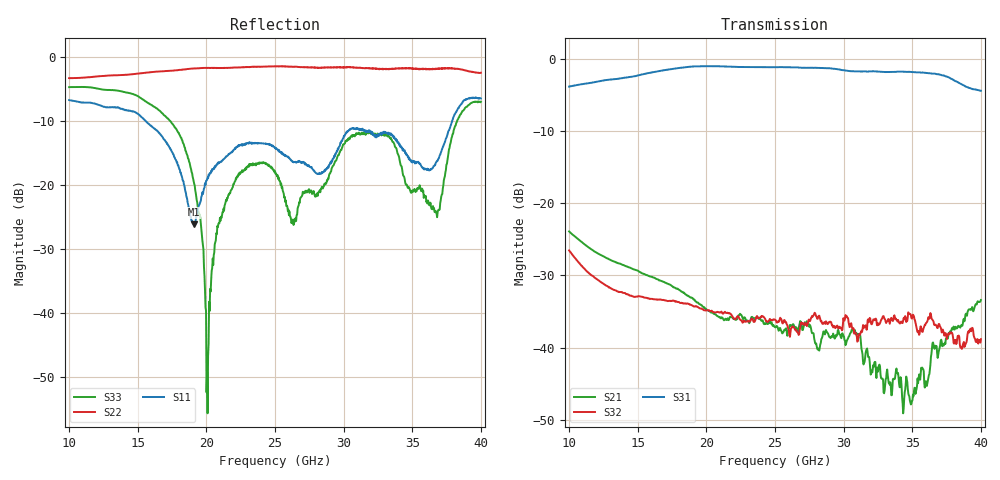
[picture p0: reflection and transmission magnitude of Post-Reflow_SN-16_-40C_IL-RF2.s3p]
!Agilent Technologies,N5245A,US49150155,A.09.90.19
!Agilent N5245A: A.09.90.19
!Date: Wednesday, November 14, 2018 00:01:03
!Correction: S11(Full 3 Port(1,2,3))
!S12(Full 3 Port(1,2,3))
!S13(Full 3 Port(1,2,3))
!S21(Full 3 Port(1,2,3))
!S22(Full 3 Port(1,2,3))
!S23(Full 3 Port(1,2,3))
!S31(Full 3 Port(1,2,3))
!S32(Full 3 Port(1,2,3))
!S33(Full 3 Port(1,2,3))
!S3P File: Measurements: <S11,S12,S13>,
!<S21,S22,S23>,
!<S31,S32,S33>:
# Hz S  dB  R 50
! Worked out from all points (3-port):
!   801 points, 10 GHz to 40 GHz, reference 50 ohm
!   strongest paths, dB at 10 GHz, 17.5 GHz, 25 GHz, 32.5 GHz, 40 GHz:
!     S31: -3.9, -1.4, -1.2, -1.8, -4.4
!     S32: -26.6, -33.5, -36.1, -36.6, -38.8
!     S21: -23.9, -31.5, -37.2, -43.3, -33.4
!   lowest |S11| = -26.2 dB at 19.11 GHz (marker M1), VSWR 1.10, Z = 45.5 - j1.2 ohm
!   |S11| at or under -10 dB: 15.59 GHz to 37.9 GHz (22.31 GHz wide, 83.4 % of centre)
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1e10  -6.70 -5.9  -23.93 59.2  -3.87 -169.8
      -23.93 59.4  -3.27 51.8  -26.57 -6.4
      -3.87 -169.6  -26.55 -6.2  -4.68 -116.9
1.49125e10  -8.70 -156.0  -29.29 -30.0  -2.38 78.0
            -29.30 -29.9  -2.58 -54.0  -32.98 -89.2
            -2.38 78.2  -32.96 -89.1  -5.99 147.9
1.91125e10  -26.15 -164.5  -33.38 -111.6  -1.08 -22.5
            -33.34 -111.5  -1.75 -126.6  -34.33 176.7
            -1.08 -22.3  -34.33 177.0  -19.79 57.9
2.00875e10  -18.81 -140.8  -34.87 -126.5  -1.05 -46.5
            -34.86 -126.5  -1.65 -138.8  -34.82 154.6
            -1.05 -46.3  -34.84 154.8  -55.68 -162.3
2.1475e10  -15.51 -159.2  -36.19 -141.2  -1.10 -80.1
           -36.19 -141.1  -1.68 -158.6  -35.25 121.5
           -1.09 -79.8  -35.20 121.6  -22.46 169.9
2.5e10  -14.24 145.8  -37.17 160.9  -1.19 -162.8
        -37.15 160.6  -1.40 153.0  -36.10 37.1
        -1.18 -162.5  -36.13 37.3  -17.80 83.1
2.905e10  -16.39 155.8  -38.69 94.9  -1.35 98.4
          -38.69 95.4  -1.62 97.2  -36.37 -62.5
          -1.35 98.8  -36.48 -61.8  -17.94 176.5
3.30625e10  -11.71 109.0  -44.36 30.9  -1.87 1.4
            -44.39 32.9  -1.89 37.3  -36.42 -153.2
            -1.86 1.9  -36.43 -153.0  -12.04 66.8
3.63625e10  -17.46 91.9  -41.34 38.0  -2.06 -87.7
            -41.29 37.7  -1.86 -17.1  -35.52 103.5
            -2.05 -87.2  -35.48 103.9  -23.35 -97.2
4e10  -6.45 69.8  -33.35 -46.3  -4.46 173.9
      -33.42 -46.3  -2.42 -75.1  -38.81 -56.2
      -4.44 174.4  -38.85 -56.2  -6.97 84.3
